|   IBIS file stm32l471_475_476_486_lqfp100.ibs
[IBIS ver]   4.2
[File name]   stm32l471_475_476_486_lqfp100.ibs
[File Rev]   4.0
[Date]   08-10-2018
[Source]   Data Created at STMicroelectronics
[Notes]   File originated from ELDO simulations.
[Disclaimer]  This information is for modeling purpose only and is
   not guaranteed.
   The information is subject to change without notice.
[Copyright]   Copyright 2018 STMicroelectronics Inc.
|   Component stm32l471_475_476_486_lqfp100
[Component] stm32l471_475_476_486_lqfp100
[Manufacturer] STMicroelectronics
[Package]
| variable   typ   min   max
R_pkg   0.0   0.0   0.0
L_pkg   0.0H   0.0H   0.0H
C_pkg   0.0F   0.0F   0.0F
[Pin]  signal_name   model_name   R_pin   L_pin   C_pin
1 PE2 io8prog2m25m50m120m_sudq_ft 132.430E-3 7.034E-9 135.000E-15
2 PE3 io8prog2m25m50m120m_sudq_ft 133.348E-3 6.765E-9 19.500E-15
3 PE4 io8prog2m25m50m120m_sudq_ft 128.973E-3 6.495E-9 10.400E-15
4 PE5 io8prog2m25m50m120m_sudq_ft 125.345E-3 6.206E-9 5.240E-15
5 PE6-WKUP io8prog2m25m50m120m_sudq_ft 120.515E-3 5.991E-9 7.820E-15
6 VBAT POWER 120.471E-3 5.950E-9 6.530E-15
7 PC13 io8prog2m25m50m120m_sudq_ft 117.881E-3 5.783E-9 6.230E-15
8 PC14-OSC32_IN io8prog2m25m50m120m_sudq_ft 117.279E-3 5.654E-9 3.110E-15
9 PC15-OSC32_OUT io8prog2m25m50m120m_sudq_ft 115.548E-3 5.548E-9 1.390E-15
10 VSS GND 114.996E-3 5.434E-9 2.920E-15
11 VDD POWER 112.976E-3 5.296E-9 3.560E-15
12 PH0-OSC_IN io8prog2m25m50m120m_sudq_ft 111.323E-3 5.231E-9 4.780E-15
13 PH1-OSC_OUT io8prog2m25m50m120m_sudq_ft 109.217E-3 5.142E-9 8.660E-15
14 NRST ioreset_ft_v33 110.664E-3 5.180E-9 9.030E-15
15 PC0 io8prog2m25m50m120m_sudq_i2c_ft 110.608E-3 5.192E-9 7.980E-15
16 PC1 io8prog2m25m50m120m_sudq_i2c_ft 111.326E-3 5.252E-9 10.300E-15
17 PC2 io8prog2m25m50m120m_sudq_ft 114.420E-3 5.345E-9 7.000E-15
18 PC3 io8prog2m25m50m120m_sudq_ft 114.363E-3 5.454E-9 8.650E-15
19 VSSA GND 117.564E-3 5.621E-9 7.825E-15
20 VREF- GND 119.905E-3 5.800E-9 229.000E-18
21 VREF+ POWER 122.312E-3 5.963E-9 1.050E-15
22 VDDA POWER 125.384E-3 6.187E-9 812.000E-18
23 PA0 io8prog2m25m50m120m_sudq_ft 129.702E-3 6.485E-9 3.820E-15
24 PA1 io8prog2m25m50m120m_sudq_ft 132.290E-3 6.715E-9 6.800E-15
25 PA2 io8prog2m25m50m120m_sudq_ft 132.955E-3 7.014E-9 16.700E-15
26 PA3 io8prog2m25m50m120m_sudq_ft 133.943E-3 7.050E-9 17.500E-15
27 VSS GND 134.958E-3 6.804E-9 12.700E-15
28 VDD POWER 130.511E-3 6.528E-9 9.830E-15
29 PA4 io8prog2m25m50m120m_sudq_ft 125.387E-3 6.245E-9 6.070E-15
30 PA5 io8prog2m25m50m120m_sudq_ft 124.989E-3 6.108E-9 577.000E-18
31 PA6 io8prog2m25m50m120m_sudq_ft 121.784E-3 5.890E-9 1.520E-15
32 PA7 io8prog2m25m50m120m_sudq_ft 119.149E-3 5.716E-9 5.440E-15
33 PC4 io8prog2m25m50m120m_sudq_ft 116.375E-3 5.556E-9 4.100E-15
34 PC5 io8prog2m25m50m120m_sudq_ft 113.279E-3 5.415E-9 3.690E-15
35 PB0 io8prog2m25m50m120m_sudq_ft 112.727E-3 5.358E-9 3.895E-15
36 PB1 io8prog2m25m50m120m_sudq_ft 112.271E-3 5.272E-9 1.660E-15
37 PB2 io8prog2m25m50m120m_sudq_ft 111.816E-3 5.238E-9 7.920E-15
38 PE7 io8prog2m25m50m120m_sudq_ft 110.999E-3 5.184E-9 9.900E-15
39 PE8 io8prog2m25m50m120m_sudq_ft 114.589E-3 5.299E-9 7.910E-15
40 PE9 io8prog2m25m50m120m_sudq_ft 114.461E-3 5.333E-9 7.940E-15
41 PE10 io8prog2m25m50m120m_sudq_ft 115.350E-3 5.424E-9 4.180E-15
42 PE11 io8prog2m25m50m120m_sudq_ft 116.979E-3 5.533E-9 6.060E-15
43 PE12 io8prog2m25m50m120m_sudq_ft 120.185E-3 5.698E-9 5.120E-15
44 PE13 io8prog2m25m50m120m_sudq_ft 122.587E-3 5.871E-9 4.740E-15
45 PE14 io8prog2m25m50m120m_sudq_ft 126.303E-3 6.069E-9 11.600E-15
46 PE15 io8prog2m25m50m120m_sudq_ft 129.715E-3 6.277E-9 9.910E-15
47 PB10 io8prog2m25m50m120m_sudq_i2c_ft 133.373E-3 6.508E-9 5.080E-15
48 PB11 io8prog2m25m50m120m_sudq_i2c_ft 137.888E-3 6.857E-9 5.470E-15
49 VSS GND 131.554E-3 6.802E-9 4.180E-15
50 VDD POWER 132.348E-3 7.042E-9 11.900E-15
51 PB12 io8w_swp_lcd4_ft 131.768E-3 7.008E-9 16.200E-15
52 PB13 io8prog2m25m50m120m_sudq_i2c_ft 131.784E-3 6.751E-9 2.150E-15
53 PB14 io8prog2m25m50m120m_sudq_i2c_ft 129.151E-3 6.483E-9 9.175E-15
54 PB15 io8prog2m25m50m120m_sudq_ft 125.191E-3 6.202E-9 5.663E-15
55 PD8 io8prog2m25m50m120m_sudq_ft 121.530E-3 5.986E-9 3.690E-15
56 PD9 io8prog2m25m50m120m_sudq_ft 118.874E-3 5.807E-9 7.430E-15
57 PD10 io8prog2m25m50m120m_sudq_ft 115.870E-3 5.635E-9 10.600E-15
58 PD11 io8prog2m25m50m120m_sudq_ft 113.226E-3 5.471E-9 5.760E-15
59 PD12 io8prog2m25m50m120m_sudq_ft 111.782E-3 5.354E-9 6.530E-15
60 PD13 io8prog2m25m50m120m_sudq_ft 110.713E-3 5.276E-9 11.400E-15
61 PD14 io8prog2m25m50m120m_sudq_ft 110.052E-3 5.204E-9 13.200E-15
62 PD15 io8prog2m25m50m120m_sudq_ft 109.954E-3 5.180E-9 14.600E-15
63 PC6 io8prog2m25m50m120m_sudq_ft 109.780E-3 5.154E-9 7.250E-15
64 PC7 io8prog2m25m50m120m_sudq_ft 112.446E-3 5.258E-9 359.000E-18
65 PC8 io8prog2m25m50m120m_sudq_ft 113.596E-3 5.332E-9 658.000E-18
66 PC9 io8prog2m25m50m120m_sudq_ft 115.707E-3 5.466E-9 508.500E-18
67 PA8 io8prog2m25m50m120m_sudq_ft 116.952E-3 5.598E-9 583.250E-18
68 PA9 POWER 119.043E-3 5.762E-9 545.875E-18
69 PA10 io8usb_id_otg20_lcd4_ft_ms 120.674E-3 5.880E-9 13.900E-15
70 PA11 io8usblsfs_otg2 124.659E-3 6.108E-9 25.000E-15
71 PA12 io8usblsfs_otg2 124.407E-3 6.161E-9 39.900E-15
72 PA13 io8prog2m25m50m120m_sudq_ft 130.156E-3 6.404E-9 302.000E-15
73 VDDUSB/VDD POWER 135.110E-3 6.824E-9 155.000E-15
74 VSS GND 139.402E-3 7.077E-9 155.000E-15
75 VDD POWER 133.554E-3 7.056E-9 39.000E-15
76 PA14 io8prog2m25m50m120m_sudq_ft 135.295E-3 7.104E-9 16.300E-15
77 PA15 io8prog2m25m50m120m_sudq_ft 132.514E-3 6.836E-9 9.760E-15
78 PC10 io8prog2m25m50m120m_sudq_ft 133.482E-3 6.641E-9 9.300E-15
79 PC11 io8prog2m25m50m120m_sudq_ft 128.366E-3 6.341E-9 5.420E-15
80 PC12 io8prog2m25m50m120m_sudq_ft 124.282E-3 6.092E-9 1.180E-15
81 PD0 io8prog2m25m50m120m_sudq_ft 121.841E-3 5.917E-9 5.460E-15
82 PD1 io8prog2m25m50m120m_sudq_ft 118.487E-3 5.728E-9 7.000E-15
83 PD2 io8prog2m25m50m120m_sudq_ft 117.180E-3 5.573E-9 6.060E-15
84 PD3 io8prog2m25m50m120m_sudq_ft 113.501E-3 5.422E-9 5.450E-15
85 PD4 io8prog2m25m50m120m_sudq_ft 113.789E-3 5.344E-9 529.000E-18
86 PD5 io8prog2m25m50m120m_sudq_ft 110.806E-3 5.256E-9 2.990E-15
87 PD6 io8prog2m25m50m120m_sudq_ft 110.442E-3 5.246E-9 2.060E-15
88 PD7 io8prog2m25m50m120m_sudq_ft 111.525E-3 5.178E-9 5.680E-15
89 PB3 io8prog2m25m50m120m_sudq_ft 111.144E-3 5.223E-9 9.910E-15
90 PB4 io8prog2m25m50m120m_sudq_ft 113.222E-3 5.310E-9 9.050E-15
91 PB5 io8prog2m25m50m120m_sudq_ft 113.323E-3 5.401E-9 12.900E-15
92 PB6 io8prog2m25m50m120m_sudq_i2c_ft 115.849E-3 5.519E-9 12.600E-15
93 PB7 io8prog2m25m50m120m_sudq_i2c_ft 117.578E-3 5.673E-9 6.140E-15
94 BOOT0 vpp_test_hv 118.982E-3 5.802E-9 9.370E-15
95 PB8 io8prog2m25m50m120m_sudq_i2c_ft 121.886E-3 5.962E-9 7.755E-15
96 PB9 io8prog2m25m50m120m_sudq_i2c_ft 126.276E-3 6.158E-9 8.563E-15
97 PE0 io8prog2m25m50m120m_sudq_ft 128.749E-3 6.367E-9 8.159E-15
98 PE1 io8prog2m25m50m120m_sudq_ft 133.288E-3 6.700E-9 1.030E-15
99 VSS GND 132.230E-3 6.844E-9 4.410E-15
100 VDD POWER 132.277E-3 7.052E-9 17.100E-15
[Model Selector] io8prog2m25m50m120m_sudq_ft
iols8p_sudq_ft_pd_lv  "IO low speed, PD=40kOhm - 1P8V"
iols8p_sudq_ft_pu_lv  "IO low speed, PU=40kOhm - 1P8V"
iols8p_sudq_ft_lv  "IO low speed - 1P8V"
iols8p_sudq_ft_pd  "IO low speed, PD=40kOhm - 3P3V"
iols8p_sudq_ft_pu  "IO low speed, PU=40kOhm - 3P3V"
iols8p_sudq_ft  "IO low speed - 3P3V"
iofs8p_sudq_ft_pd_lv  "IO full speed, PD=40kOhm - 1P8V"
iofs8p_sudq_ft_pu_lv  "IO full speed, PU=40kOhm - 1P8V"
iofs8p_sudq_ft_lv  "IO full speed - 1P8V"
iofs8p_sudq_ft_pd  "IO full speed, PD=40kOhm - 3P3V"
iofs8p_sudq_ft_pu  "IO full speed, PU=40kOhm - 3P3V"
iofs8p_sudq_ft  "IO full speed - 3P3V"
ioms8p_sudq_ft_pd_lv  "IO medium speed, PD=40kOhm - 1P8V"
ioms8p_sudq_ft_pu_lv  "IO medium speed, PU=40kOhm - 1P8V"
ioms8p_sudq_ft_lv  "IO medium speed - 1P8V"
ioms8p_sudq_ft_pd  "IO medium speed, PD=40kOhm - 3P3V"
ioms8p_sudq_ft_pu  "IO medium speed, PU=40kOhm - 3P3V"
ioms8p_sudq_ft  "IO medium speed - 3P3V"
iohs8p_sudq_ft_pd_lv  "IO high speed, PD=40kOhm - 1P8V"
iohs8p_sudq_ft_pu_lv  "IO high speed, PU=40kOhm - 1P8V"
iohs8p_sudq_ft_lv  "IO high speed - 1P8V"
iohs8p_sudq_ft_pd  "IO high speed, PD=40kOhm - 3P3V"
iohs8p_sudq_ft_pu  "IO high speed, PU=40kOhm - 3P3V"
iohs8p_sudq_ft  "IO high speed - 3P3V"
[Model Selector] io8prog2m25m50m120m_sudq_i2c_ft
io8prog_1v8_i2c_pd  "5V Tol GPIO 1.8V range i2c functionality with pull down"
io8prog_1v8_i2c_pu  "5V Tol GPIO 1.8V range i2c functionality with pull up"
io8prog_1v8_i2c  "5V Tol GPIO 1.8V range i2c functionality"
io8prog_3v3_i2c_pd  "5V Tol GPIO 3.3V range i2c functionality with pull down"
io8prog_3v3_i2c_pu  "5V Tol GPIO 3.3V range i2c functionality with pull up"
io8prog_3v3_i2c  "5V Tol GPIO 3.3V range i2c functionality"
io8ls_1v8_pd  "5V Tol GPIO 1.8V range with pd io low speed"
io8ls_1v8_pu  "5V Tol GPIO 1.8V range with pu io low speed"
io8ls_1v8  "5V Tol GPIO 1.8V range io low speed"
io8ls_3v3_pd  "5V Tol GPIO 3.3V range with pd io low speed"
io8ls_3v3_pu  "5V Tol GPIO 3.3V range with pu io low speed"
io8ls_3v3  "5V Tol GPIO 3.3V range io low speed"
io8fs_1v8_pd  "5V Tol GPIO 1.8V range with pd io full speed"
io8fs_1v8_pu  "5V Tol GPIO 1.8V range with pu io full speed"
io8fs_1v8  "5V Tol GPIO 1.8V range io full speed"
io8fs_3v3_pd  "5V Tol GPIO 3.3V range with pd io full speed"
io8fs_3v3_pu  "5V Tol GPIO 3.3V range with pu io full speed"
io8fs_3v3  "5V Tol GPIO 3.3V range io full speed"
io8ms_1v8_pd  "5V Tol GPIO 1.8V range with pd io medium speed"
io8ms_1v8_pu  "5V Tol GPIO 1.8V range with pu io medium speed"
io8ms_1v8  "5V Tol GPIO 1.8V range io medium speed"
io8ms_3v3_pd  "5V Tol GPIO 3.3V range with pd io medium speed"
io8ms_3v3_pu  "5V Tol GPIO 3.3V range with pu io medium speed"
io8ms_3v3  "5V Tol GPIO 3.3V range io medium speed"
io8hs_1v8_pd  "5V Tol GPIO 1.8V range with pd io high speed"
io8hs_1v8_pu  "5V Tol GPIO 1.8V range with pu io high speed"
io8hs_1v8  "5V Tol GPIO 1.8V range io high speed"
io8hs_3v3_pd  "5V Tol GPIO 3.3V range with pd io high speed"
io8hs_3v3_pu  "5V Tol GPIO 3.3V range with pu io high speed"
io8hs_3v3  "5V Tol GPIO 3.3V range io high speed"
[Model Selector] io8usb_id_otg20_lcd4_ft_ms
io8usbid_1v8_id_pu  "ID 1V8 range with pull up"
io8usbid_3v3_id_pu  "ID 3V3 range with pull up"
io8usbid_1v8_id  "ID 1V8 range"
io8usbid_3v3_id  "ID 3V3 range"
io8lsusbid_1v8_pd  "GPIO 1.8V range with pd io low speed"
io8lsusbid_1v8_pu  "GPIO 1.8V range with pu io low speed"
io8lsusbid_1v8  "GPIO 1.8V range io low speed"
io8lsusbid_3v3_pd  "GPIO 3.3V range with pd io low speed"
io8lsusbid_3v3_pu  "GPIO 3.3V range with pu io low speed"
io8lsusbid_3v3  "GPIO 3.3V range io low speed"
io8fsusbid_1v8_pd  "GPIO 1.8V range with pd io full speed"
io8fsusbid_1v8_pu  "GPIO 1.8V range with pu io full speed"
io8fsusbid_1v8  "GPIO 1.8V range io full speed"
io8fsusbid_3v3_pd  "GPIO 3.3V range with pd io full speed"
io8fsusbid_3v3_pu  "GPIO 3.3V range with pu io full speed"
io8fsusbid_3v3  "GPIO 3.3V range io full speed"
io8msusbid_1v8_pd  "GPIO 1.8V range with pd io medium speed"
io8msusbid_1v8_pu  "GPIO 1.8V range with pu io medium speed"
io8msusbid_1v8  "GPIO 1.8V range io medium speed"
io8msusbid_3v3_pd  "GPIO 3.3V range with pd io medium speed"
io8msusbid_3v3_pu  "GPIO 3.3V range with pu io medium speed"
io8msusbid_3v3  "GPIO 3.3V range io medium speed"
io8hsusbid_1v8_pd  "GPIO 1.8V range with pd io high speed"
io8hsusbid_1v8_pu  "GPIO 1.8V range with pu io high speed"
io8hsusbid_1v8  "GPIO 1.8V range io high speed"
io8hsusbid_3v3_pd  "GPIO 3.3V range with pd io high speed"
io8hsusbid_3v3_pu  "GPIO 3.3V range with pu io high speed"
io8hsusbid_3v3  "GPIO 3.3V range io high speed"
[Model Selector] io8usblsfs_otg2
usb_ls_pd  "USB Low Speed mode - Pull Down"
usb_ls_pu2  "USB Low Speed mode - Pull up 2"
usb_ls_pu  "USB Low Speed mode - Pull up"
usb_fs  "USB Low Speed mode"
usb_fs_pd  "USB Full Speed mode - Pull Down"
usb_fs_pu2  "USB Full Speed mode - Pull up 2"
usb_fs_pu  "USB Full Speed mode - Pull up"
[Model Selector] ioreset_ft_v33
ioreset_1v2_pu  "RESET 1.2V range with PU"
ioreset_1v2  "RESET 1.2V range"
ioreset_1v8_pu  "RESET 1.8V range with PU"
ioreset_1v8  "RESET 1.8V range"
ioreset_3v3_pu  "RESET 3.3V range with PU"
ioreset_3v3  "RESET 3.3V range"
[Model Selector] io8w_swp_lcd4_ft
io8w_swp_classc  "Class C swp functionality"
io8w_swp_classb  "Class B swp functionality"
io8lsw_1v8_pd  "GPIO 1.8V range with pd io low speed"
io8lsw_1v8_pu  "GPIO 1.8V range with pu io low speed"
io8lsw_1v8  "GPIO 1.8V range io low speed"
io8lsw_3v3_pd  "GPIO 3.3V range with pd io low speed"
io8lsw_3v3_pu  "GPIO 3.3V range with pu io low speed"
io8lsw_3v3  "GPIO 3.3V range io low speed"
io8fsw_1v8_pd  "GPIO 1.8V range with pd io full speed"
io8fsw_1v8_pu  "GPIO 1.8V range with pu io full speed"
io8fsw_1v8  "GPIO 1.8V range io full speed"
io8fsw_3v3_pd  "GPIO 3.3V range with pd io full speed"
io8fsw_3v3_pu  "GPIO 3.3V range with pu io full speed"
io8fsw_3v3  "GPIO 3.3V range io full speed"
io8msw_1v8_pd  "GPIO 1.8V range with pd io medium speed"
io8msw_1v8_pu  "GPIO 1.8V range with pu io medium speed"
io8msw_1v8  "GPIO 1.8V range io medium speed"
io8msw_3v3_pd  "GPIO 3.3V range with pd io medium speed"
io8msw_3v3_pu  "GPIO 3.3V range with pu io medium speed"
io8msw_3v3  "GPIO 3.3V range io medium speed"
io8hsw_1v8_pd  "GPIO 1.8V range with pd io high speed"
io8hsw_1v8_pu  "GPIO 1.8V range with pu io high speed"
io8hsw_1v8  "GPIO 1.8V range io high speed"
io8hsw_3v3_pd  "GPIO 3.3V range with pd io high speed"
io8hsw_3v3_pu  "GPIO 3.3V range with pu io high speed"
io8hsw_3v3  "GPIO 3.3V range io high speed"
[Model Selector] vpp_test_hv
vpp_1v8  "VPP with test functionality 1.8V range"
vpp_3v3  "VPP with test functionality 3.3V range"
| Models and submodels in the file (123): iols8p_sudq_ft_pd_lv (I/O), iols8p_sudq_ft_pu_lv (I/O), iols8p_sudq_ft_lv (I/O), iols8p_sudq_ft_pd (I/O), iols8p_sudq_ft_pu (I/O), iols8p_sudq_ft (I/O), iofs8p_sudq_ft_pd_lv (I/O), iofs8p_sudq_ft_pu_lv (I/O), iofs8p_sudq_ft_lv (I/O), iofs8p_sudq_ft_pd (I/O), iofs8p_sudq_ft_pu (I/O), iofs8p_sudq_ft (I/O), ioms8p_sudq_ft_pd_lv (I/O), ioms8p_sudq_ft_pu_lv (I/O), ioms8p_sudq_ft_lv (I/O), ioms8p_sudq_ft_pd (I/O), ioms8p_sudq_ft_pu (I/O), ioms8p_sudq_ft (I/O), iohs8p_sudq_ft_pd_lv (I/O), iohs8p_sudq_ft_pu_lv (I/O), iohs8p_sudq_ft_lv (I/O), iohs8p_sudq_ft_pd (I/O), iohs8p_sudq_ft_pu (I/O), iohs8p_sudq_ft (I/O), io8prog_1v8_i2c_pd (I/O), io8prog_1v8_i2c_pu (I/O), io8prog_1v8_i2c (I/O), io8prog_3v3_i2c_pd (I/O), io8prog_3v3_i2c_pu (I/O), io8prog_3v3_i2c (I/O), io8ls_1v8_pd (I/O), io8ls_1v8_pu (I/O), io8ls_1v8 (I/O), io8ls_3v3_pd (I/O), io8ls_3v3_pu (I/O), io8ls_3v3 (I/O), io8fs_1v8_pd (I/O), io8fs_1v8_pu (I/O), io8fs_1v8 (I/O), io8fs_3v3_pd (I/O), io8fs_3v3_pu (I/O), io8fs_3v3 (I/O), io8ms_1v8_pd (I/O), io8ms_1v8_pu (I/O), io8ms_1v8 (I/O), io8ms_3v3_pd (I/O), io8ms_3v3_pu (I/O), io8ms_3v3 (I/O), io8hs_1v8_pd (I/O), io8hs_1v8_pu (I/O), io8hs_1v8 (I/O), io8hs_3v3_pd (I/O), io8hs_3v3_pu (I/O), io8hs_3v3 (I/O), io8usbid_1v8_id_pu (Input), io8usbid_3v3_id_pu (Input), io8usbid_1v8_id (Input), io8usbid_3v3_id (Input), io8lsusbid_1v8_pd (I/O), io8lsusbid_1v8_pu (I/O), io8lsusbid_1v8 (I/O), io8lsusbid_3v3_pd (I/O), io8lsusbid_3v3_pu (I/O), io8lsusbid_3v3 (I/O), io8fsusbid_1v8_pd (I/O), io8fsusbid_1v8_pu (I/O), io8fsusbid_1v8 (I/O), io8fsusbid_3v3_pd (I/O), io8fsusbid_3v3_pu (I/O), io8fsusbid_3v3 (I/O), io8msusbid_1v8_pd (I/O), io8msusbid_1v8_pu (I/O), io8msusbid_1v8 (I/O), io8msusbid_3v3_pd (I/O), io8msusbid_3v3_pu (I/O), io8msusbid_3v3 (I/O), io8hsusbid_1v8_pd (I/O), io8hsusbid_1v8_pu (I/O), io8hsusbid_1v8 (I/O), io8hsusbid_3v3_pd (I/O)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
